TYPE Alarm :
STRUCT
	PRESSURE:BOOL;
	MFC1:BOOL;
	WALL_TEMP:BOOL;
	LID_TEMP:BOOL;
	STAGE_TEMP1:BOOL;
	STAGE_TEMP2:BOOL;
	STAGE_TEMP3:BOOL;
	STAGE_TEMP4:BOOL;
	Gas1FlowPressureOutOfRange:BOOL;
	TurboN2PurgePressureOutOfRange:BOOL;
	PrepareTransferTimerout:BOOL;
	TransferWaferTimeout:BOOL;
	OpenGasValveTimeout:BOOL;
	CloseGasValveTimeout:BOOL;
	OpenCloseSlitValveTimeout:BOOL;
	ATMCheckTimeout:BOOL;
	
	PLC:BOOL;	
	DRY_PUMP:BOOL;
	PENDULUM_VALVE:BOOL;
	TURBO_PUMP:BOOL;	
	//PROCESS TOLERANCE
	TOLERANCE_PRESSURE:BOOL;
	TOLERANCE_MFC1:BOOL;
	TOLERANCE_WALL_TEMP:BOOL;
	TOLERANCE_LID_TEMP:BOOL;
	TOLERANCE_STAGE_TEMP1,
	TOLERANCE_STAGE_TEMP2,
	TOLERANCE_STAGE_TEMP3,
	TOLERANCE_STAGE_TEMP4: BOOL;


END_STRUCT
END_TYPE
